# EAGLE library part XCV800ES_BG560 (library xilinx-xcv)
xcv800es_bg560 edit this description Auto generated by make-symbol-device-package-bsdl.ulp Rev. 26 Source: xcv800es_bg560.bsd
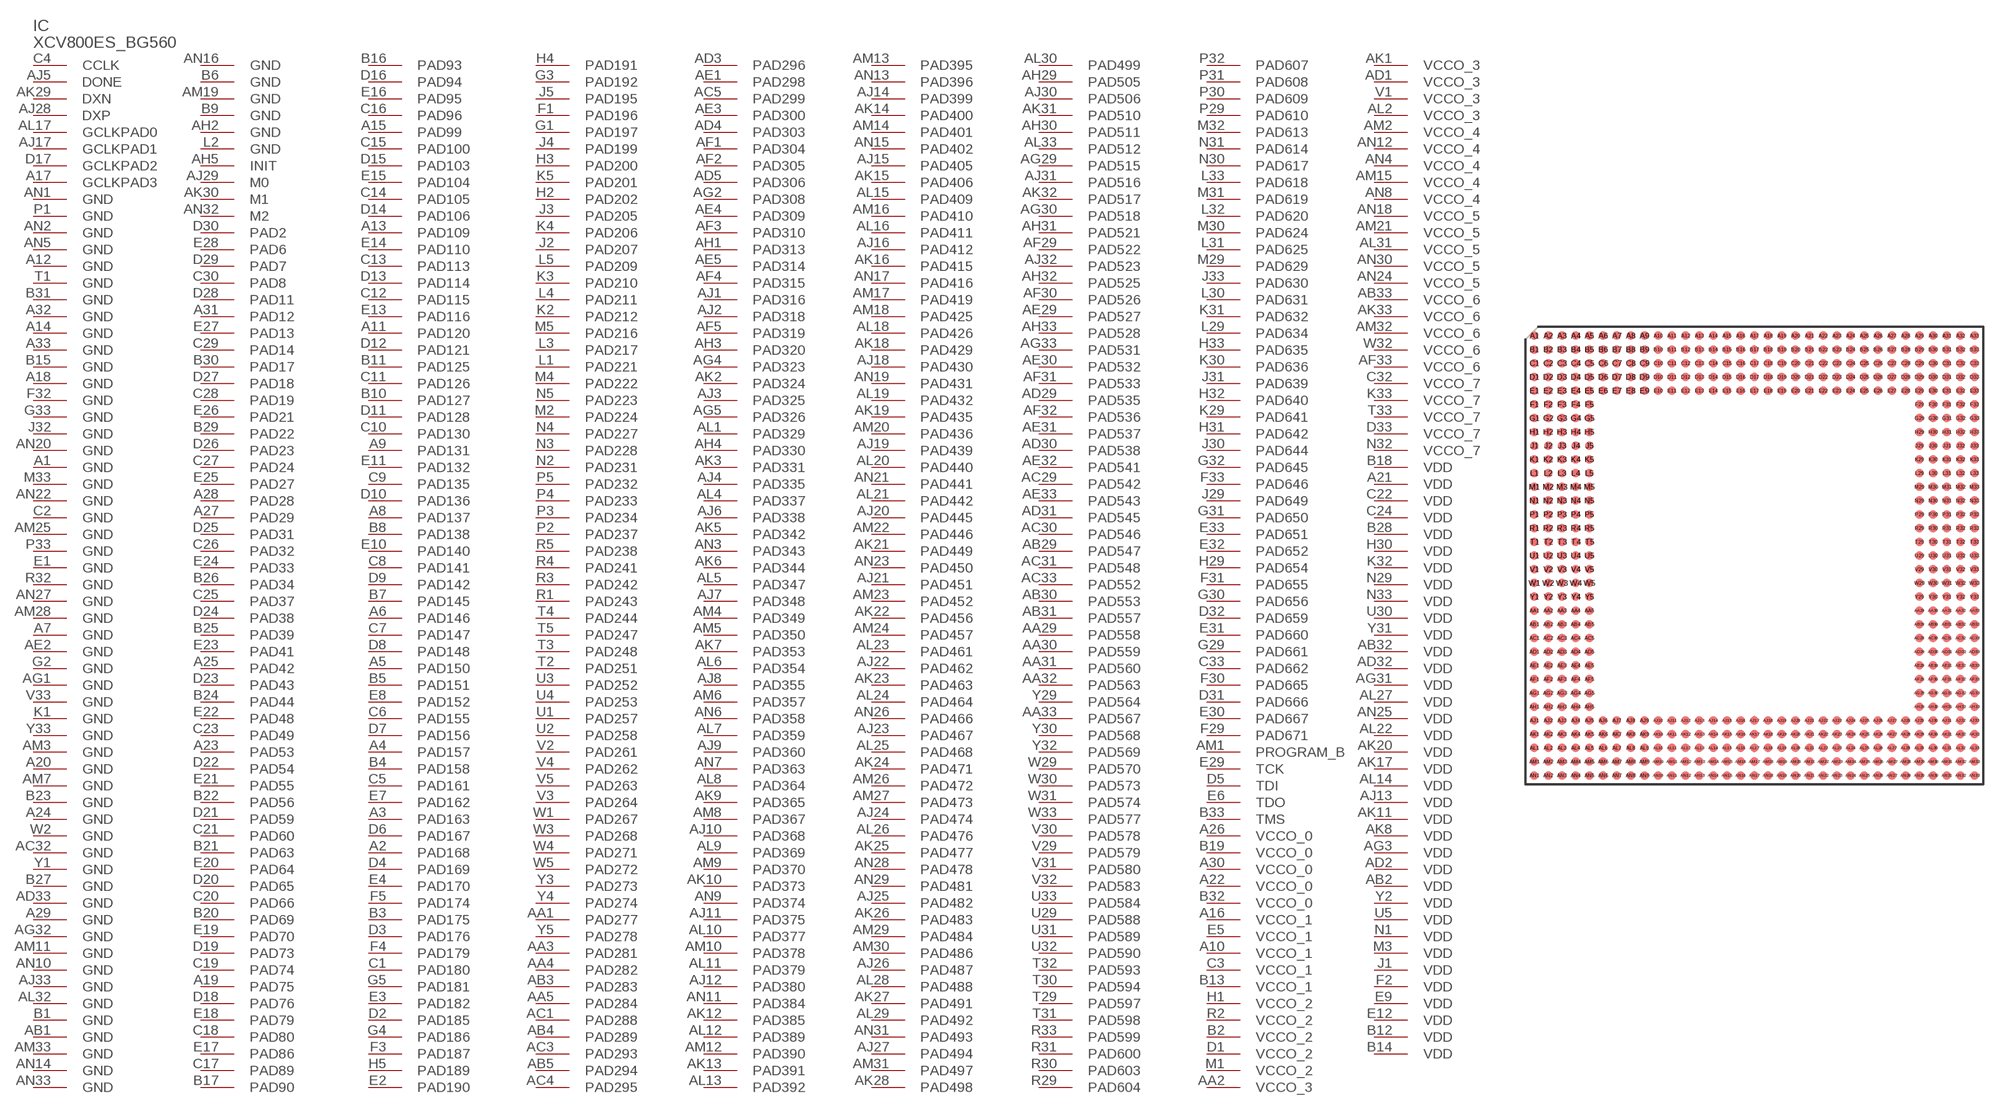
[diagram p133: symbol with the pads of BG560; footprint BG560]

Designator prefix IC

## XCV800ES_BG560 (OC_FARNELL: unknown; OC_NEWARK: unknown)  [BG560]
A1  GND  pwr
A2  PAD168
A3  PAD163
A4  PAD157
A5  PAD150
A6  PAD146
A7  GND  pwr
A8  PAD137
A9  PAD131
A10  VCCO_1  pwr
A11  PAD120
A12  GND  pwr
A13  PAD109
A14  GND  pwr
A15  PAD99
A16  VCCO_1  pwr
A17  GCLKPAD3  in
A18  GND  pwr
A19  PAD75
A20  GND  pwr
A21  VDD  pwr
A22  VCCO_0  pwr
A23  PAD53
A24  GND  pwr
A25  PAD42
A26  VCCO_0  pwr
A27  PAD29
A28  PAD28
A29  GND  pwr
A30  VCCO_0  pwr
A31  PAD12
A32  GND  pwr
A33  GND  pwr
AA1  PAD277
AA2  VCCO_3  pwr
AA3  PAD281
AA4  PAD282
AA5  PAD284
AA29  PAD558
AA30  PAD559
AA31  PAD560
AA32  PAD563
AA33  PAD567
AB1  GND  pwr
AB2  VDD  pwr
AB3  PAD283
AB4  PAD289
AB5  PAD294
AB29  PAD547
AB30  PAD553
AB31  PAD557
AB32  VDD  pwr
AB33  VCCO_6  pwr
AC1  PAD288
AC3  PAD293
AC4  PAD295
AC5  PAD299
AC29  PAD542
AC30  PAD546
AC31  PAD548
AC32  GND  pwr
AC33  PAD552
AD1  VCCO_3  pwr
AD2  VDD  pwr
AD3  PAD296
AD4  PAD303
AD5  PAD306
AD29  PAD535
AD30  PAD538
AD31  PAD545
AD32  VDD  pwr
AD33  GND  pwr
AE1  PAD298
AE2  GND  pwr
AE3  PAD300
AE4  PAD309
AE5  PAD314
AE29  PAD527
AE30  PAD532
AE31  PAD537
AE32  PAD541
AE33  PAD543
AF1  PAD304
AF2  PAD305
AF3  PAD310
AF4  PAD315
AF5  PAD319
AF29  PAD522
AF30  PAD526
AF31  PAD533
AF32  PAD536
AF33  VCCO_6  pwr
AG1  GND  pwr
AG2  PAD308
AG3  VDD  pwr
AG4  PAD323
AG5  PAD326
AG29  PAD515
AG30  PAD518
AG31  VDD  pwr
AG32  GND  pwr
AG33  PAD531
AH1  PAD313
AH2  GND  pwr
AH3  PAD320
AH4  PAD330
AH5  INIT
AH29  PAD505
AH30  PAD511
AH31  PAD521
AH32  PAD525
AH33  PAD528
AJ1  PAD316
AJ2  PAD318
AJ3  PAD325
AJ4  PAD335
AJ5  DONE
AJ6  PAD338
AJ7  PAD348
AJ8  PAD355
AJ9  PAD360
AJ10  PAD368
AJ11  PAD375
AJ12  PAD380
AJ13  VDD  pwr
AJ14  PAD399
AJ15  PAD405
AJ16  PAD412
AJ17  GCLKPAD1  in
AJ18  PAD430
AJ19  PAD439
AJ20  PAD445
AJ21  PAD451
AJ22  PAD462
AJ23  PAD467
AJ24  PAD474
AJ25  PAD482
AJ26  PAD487
AJ27  PAD494
AJ28  DXP  pas
AJ29  M0  in
AJ30  PAD506
AJ31  PAD516
AJ32  PAD523
AJ33  GND  pwr
AK1  VCCO_3  pwr
AK2  PAD324
AK3  PAD331
AK5  PAD342
AK6  PAD344
AK7  PAD353
AK8  VDD  pwr
AK9  PAD365
AK10  PAD373
AK11  VDD  pwr
AK12  PAD385
AK13  PAD391
AK14  PAD400
AK15  PAD406
AK16  PAD415
AK17  VDD  pwr
AK18  PAD429
AK19  PAD435
AK20  VDD  pwr
AK21  PAD449
AK22  PAD456
AK23  PAD463
AK24  PAD471
AK25  PAD477
AK26  PAD483
AK27  PAD491
AK28  PAD498
AK29  DXN  pas
AK30  M1  in
AK31  PAD510
AK32  PAD517
AK33  VCCO_6  pwr
AL1  PAD329
AL2  VCCO_3  pwr
AL4  PAD337
AL5  PAD347
AL6  PAD354
AL7  PAD359
AL8  PAD364
AL9  PAD369
AL10  PAD377
AL11  PAD379
AL12  PAD389
AL13  PAD392
AL14  VDD  pwr
AL15  PAD409
AL16  PAD411
AL17  GCLKPAD0  in
AL18  PAD426
AL19  PAD432
AL20  PAD440
AL21  PAD442
AL22  VDD  pwr
AL23  PAD461
AL24  PAD464
AL25  PAD468
AL26  PAD476
AL27  VDD  pwr
AL28  PAD488
AL29  PAD492
AL30  PAD499
AL31  VCCO_5  pwr
AL32  GND  pwr
AL33  PAD512
AM1  PROGRAM_B  in
AM2  VCCO_4  pwr
AM3  GND  pwr
AM4  PAD349
AM5  PAD350
AM6  PAD357
AM7  GND  pwr
AM8  PAD367
AM9  PAD370
AM10  PAD378
AM11  GND  pwr
AM12  PAD390
AM13  PAD395
AM14  PAD401
AM15  VCCO_4  pwr
AM16  PAD410
AM17  PAD419
AM18  PAD425
AM19  GND  pwr
AM20  PAD436
AM21  VCCO_5  pwr
AM22  PAD446
AM23  PAD452
AM24  PAD457
AM25  GND  pwr
AM26  PAD472
AM27  PAD473
AM28  GND  pwr
AM29  PAD484
AM30  PAD486
AM31  PAD497
AM32  VCCO_6  pwr
AM33  GND  pwr
AN1  GND  pwr
AN2  GND  pwr
AN3  PAD343
AN4  VCCO_4  pwr
AN5  GND  pwr
AN6  PAD358
AN7  PAD363
AN8  VCCO_4  pwr
AN9  PAD374
AN10  GND  pwr
AN11  PAD384
AN12  VCCO_4  pwr
AN13  PAD396
AN14  GND  pwr
AN15  PAD402
AN16  GND  pwr
AN17  PAD416
AN18  VCCO_5  pwr
AN19  PAD431
AN20  GND  pwr
AN21  PAD441
AN22  GND  pwr
AN23  PAD450
AN24  VCCO_5  pwr
AN25  VDD  pwr
AN26  PAD466
AN27  GND  pwr
AN28  PAD478
AN29  PAD481
AN30  VCCO_5  pwr
AN31  PAD493
AN32  M2  in
AN33  GND  pwr
B1  GND  pwr
B2  VCCO_2  pwr
B3  PAD175
B4  PAD158
B5  PAD151
B6  GND  pwr
B7  PAD145
B8  PAD138
B9  GND  pwr
B10  PAD127
B11  PAD125
B12  VDD  pwr
B13  VCCO_1  pwr
B14  VDD  pwr
B15  GND  pwr
B16  PAD93
B17  PAD90
B18  VDD  pwr
B19  VCCO_0  pwr
B20  PAD69
B21  PAD63
B22  PAD56
B23  GND  pwr
B24  PAD44
B25  PAD39
B26  PAD34
B27  GND  pwr
B28  VDD  pwr
B29  PAD22
B30  PAD17
B31  GND  pwr
B32  VCCO_0  pwr
B33  TMS  in
C1  PAD180
C2  GND  pwr
C3  VCCO_1  pwr
C4  CCLK
C5  PAD161
C6  PAD155
C7  PAD147
C8  PAD141
C9  PAD135
C10  PAD130
C11  PAD126
C12  PAD115
C13  PAD113
C14  PAD105
C15  PAD100
C16  PAD96
C17  PAD89
C18  PAD80
C19  PAD74
C20  PAD66
C21  PAD60
C22  VDD  pwr
C23  PAD49
C24  VDD  pwr
C25  PAD37
C26  PAD32
C27  PAD24
C28  PAD19
C29  PAD14
C30  PAD8
C32  VCCO_7  pwr
C33  PAD662
D1  VCCO_2  pwr
D2  PAD185
D3  PAD176
D4  PAD169
D5  TDI  in
D6  PAD167
D7  PAD156
D8  PAD148
D9  PAD142
D10  PAD136
D11  PAD128
D12  PAD121
D13  PAD114
D14  PAD106
D15  PAD103
D16  PAD94
D17  GCLKPAD2  in
D18  PAD76
D19  PAD73
D20  PAD65
D21  PAD59
D22  PAD54
D23  PAD43
D24  PAD38
D25  PAD31
D26  PAD23
D27  PAD18
D28  PAD11
D29  PAD7
D30  PAD2
D31  PAD666
D32  PAD659
D33  VCCO_7  pwr
E1  GND  pwr
E2  PAD190
E3  PAD182
E4  PAD170
E5  VCCO_1  pwr
E6  TDO  out
E7  PAD162
E8  PAD152
E9  VDD  pwr
E10  PAD140
E11  PAD132
E12  VDD  pwr
E13  PAD116
E14  PAD110
E15  PAD104
E16  PAD95
E17  PAD86
E18  PAD79
E19  PAD70
E20  PAD64
E21  PAD55
E22  PAD48
E23  PAD41
E24  PAD33
E25  PAD27
E26  PAD21
E27  PAD13
E28  PAD6
E29  TCK  in
E30  PAD667
E31  PAD660
E32  PAD652
E33  PAD651
F1  PAD196
F2  VDD  pwr
F3  PAD187
F4  PAD179
F5  PAD174
F29  PAD671
F30  PAD665
F31  PAD655
F32  GND  pwr
F33  PAD646
G1  PAD197
G2  GND  pwr
G3  PAD192
G4  PAD186
G5  PAD181
G29  PAD661
G30  PAD656
G31  PAD650
G32  PAD645
G33  GND  pwr
H1  VCCO_2  pwr
H2  PAD202
H3  PAD200
H4  PAD191
H5  PAD189
H29  PAD654
H30  VDD  pwr
H31  PAD642
H32  PAD640
H33  PAD635
J1  VDD  pwr
J2  PAD207
J3  PAD205
J4  PAD199
J5  PAD195
J29  PAD649
J30  PAD644
J31  PAD639
J32  GND  pwr
J33  PAD630
K1  GND  pwr
K2  PAD212
K3  PAD210
K4  PAD206
K5  PAD201
K29  PAD641
K30  PAD636
K31  PAD632
K32  VDD  pwr
K33  VCCO_7  pwr
L1  PAD221
L2  GND  pwr
L3  PAD217
L4  PAD211
L5  PAD209
L29  PAD634
L30  PAD631
L31  PAD625
L32  PAD620
L33  PAD618
M1  VCCO_2  pwr
M2  PAD224
M3  VDD  pwr
M4  PAD222
M5  PAD216
M29  PAD629
M30  PAD624
M31  PAD619
M32  PAD613
M33  GND  pwr
N1  VDD  pwr
N2  PAD231
N3  PAD228
N4  PAD227
N5  PAD223
N29  VDD  pwr
N30  PAD617
N31  PAD614
N32  VCCO_7  pwr
N33  VDD  pwr
P1  GND  pwr
P2  PAD237
P3  PAD234
P4  PAD233
P5  PAD232
P29  PAD610
P30  PAD609
P31  PAD608
P32  PAD607
P33  GND  pwr
R1  PAD243
R2  VCCO_2  pwr
R3  PAD242
R4  PAD241
R5  PAD238
R29  PAD604
R30  PAD603
R31  PAD600
R32  GND  pwr
R33  PAD599
T1  GND  pwr
T2  PAD251
T3  PAD248
T4  PAD244
T5  PAD247
T29  PAD597
T30  PAD594
T31  PAD598
T32  PAD593
T33  VCCO_7  pwr
U1  PAD257
U2  PAD258
U3  PAD252
U4  PAD253
U5  VDD  pwr
U29  PAD588
U30  VDD  pwr
U31  PAD589
U32  PAD590
U33  PAD584
V1  VCCO_3  pwr
V2  PAD261
V3  PAD264
V4  PAD262
V5  PAD263
V29  PAD579
V30  PAD578
V31  PAD580
V32  PAD583
V33  GND  pwr
W1  PAD267
W2  GND  pwr
W3  PAD268
W4  PAD271
W5  PAD272
W29  PAD570
W30  PAD573
W31  PAD574
W32  VCCO_6  pwr
W33  PAD577
Y1  GND  pwr
Y2  VDD  pwr
Y3  PAD273
Y4  PAD274
Y5  PAD278
Y29  PAD564
Y30  PAD568
Y31  VDD  pwr
Y32  PAD569
Y33  GND  pwr

## Footprint BG560 (pad centres in mm)
Metal BGA (BG560) Auto generated by make-symbol-device-package-bsdl.ulp Rev. 26 Source: xcv1000_bg560_1532.bsd; bg560.pdf
smd 0.8 x 0.8: A1 -20.32,20.32; A2 -19.05,20.32; A3 -17.78,20.32; A4 -16.51,20.32; A5 -15.24,20.32; A6 -13.97,20.32; A7 -12.7,20.32; A8 -11.43,20.32; A9 -10.16,20.32; A10 -8.89,20.32; A11 -7.62,20.32; A12 -6.35,20.32; A13 -5.08,20.32; A14 -3.81,20.32; A15 -2.54,20.32; A16 -1.27,20.32; A17 0,20.32; A18 1.27,20.32; A19 2.54,20.32; A20 3.81,20.32; A21 5.08,20.32; A22 6.35,20.32; A23 7.62,20.32; A24 8.89,20.32; A25 10.16,20.32; A26 11.43,20.32; A27 12.7,20.32; A28 13.97,20.32; A29 15.24,20.32; A30 16.51,20.32; A31 17.78,20.32; A32 19.05,20.32; A33 20.32,20.32; AA1 -20.32,-5.08; AA2 -19.05,-5.08; AA3 -17.78,-5.08; AA4 -16.51,-5.08; AA5 -15.24,-5.08; AA29 15.24,-5.08; AA30 16.51,-5.08; AA31 17.78,-5.08; AA32 19.05,-5.08; AA33 20.32,-5.08; AB1 -20.32,-6.35; AB2 -19.05,-6.35; AB3 -17.78,-6.35; AB4 -16.51,-6.35; AB5 -15.24,-6.35; AB29 15.24,-6.35; AB30 16.51,-6.35; AB31 17.78,-6.35; AB32 19.05,-6.35; AB33 20.32,-6.35; AC1 -20.32,-7.62; AC2 -19.05,-7.62; AC3 -17.78,-7.62; AC4 -16.51,-7.62; AC5 -15.24,-7.62; AC29 15.24,-7.62; AC30 16.51,-7.62; AC31 17.78,-7.62; AC32 19.05,-7.62; AC33 20.32,-7.62; AD1 -20.32,-8.89; AD2 -19.05,-8.89; AD3 -17.78,-8.89; AD4 -16.51,-8.89; AD5 -15.24,-8.89; AD29 15.24,-8.89; AD30 16.51,-8.89; AD31 17.78,-8.89; AD32 19.05,-8.89; AD33 20.32,-8.89; AE1 -20.32,-10.16; AE2 -19.05,-10.16; AE3 -17.78,-10.16; AE4 -16.51,-10.16; AE5 -15.24,-10.16; AE29 15.24,-10.16; AE30 16.51,-10.16; AE31 17.78,-10.16; AE32 19.05,-10.16; AE33 20.32,-10.16; AF1 -20.32,-11.43; AF2 -19.05,-11.43; AF3 -17.78,-11.43; AF4 -16.51,-11.43; AF5 -15.24,-11.43; AF29 15.24,-11.43; AF30 16.51,-11.43; AF31 17.78,-11.43; AF32 19.05,-11.43; AF33 20.32,-11.43; AG1 -20.32,-12.7; AG2 -19.05,-12.7; AG3 -17.78,-12.7; AG4 -16.51,-12.7; AG5 -15.24,-12.7; AG29 15.24,-12.7; AG30 16.51,-12.7; AG31 17.78,-12.7; AG32 19.05,-12.7; AG33 20.32,-12.7; AH1 -20.32,-13.97; AH2 -19.05,-13.97; AH3 -17.78,-13.97; AH4 -16.51,-13.97; AH5 -15.24,-13.97; AH29 15.24,-13.97; AH30 16.51,-13.97; AH31 17.78,-13.97; AH32 19.05,-13.97; AH33 20.32,-13.97; AJ1 -20.32,-15.24; AJ2 -19.05,-15.24; AJ3 -17.78,-15.24; AJ4 -16.51,-15.24; AJ5 -15.24,-15.24; AJ6 -13.97,-15.24; AJ7 -12.7,-15.24; AJ8 -11.43,-15.24; AJ9 -10.16,-15.24; AJ10 -8.89,-15.24; AJ11 -7.62,-15.24; AJ12 -6.35,-15.24; AJ13 -5.08,-15.24; AJ14 -3.81,-15.24; AJ15 -2.54,-15.24; AJ16 -1.27,-15.24; AJ17 0,-15.24; AJ18 1.27,-15.24; AJ19 2.54,-15.24; AJ20 3.81,-15.24; AJ21 5.08,-15.24; AJ22 6.35,-15.24; AJ23 7.62,-15.24; AJ24 8.89,-15.24; AJ25 10.16,-15.24; AJ26 11.43,-15.24; AJ27 12.7,-15.24; AJ28 13.97,-15.24; AJ29 15.24,-15.24; AJ30 16.51,-15.24; AJ31 17.78,-15.24; AJ32 19.05,-15.24; AJ33 20.32,-15.24; AK1 -20.32,-16.51; AK2 -19.05,-16.51; AK3 -17.78,-16.51; AK4 -16.51,-16.51; AK5 -15.24,-16.51; AK6 -13.97,-16.51; AK7 -12.7,-16.51; AK8 -11.43,-16.51; AK9 -10.16,-16.51; AK10 -8.89,-16.51; AK11 -7.62,-16.51; AK12 -6.35,-16.51; AK13 -5.08,-16.51; AK14 -3.81,-16.51; AK15 -2.54,-16.51; AK16 -1.27,-16.51; AK17 0,-16.51; AK18 1.27,-16.51; AK19 2.54,-16.51; AK20 3.81,-16.51; AK21 5.08,-16.51; AK22 6.35,-16.51; AK23 7.62,-16.51; AK24 8.89,-16.51; AK25 10.16,-16.51; AK26 11.43,-16.51; AK27 12.7,-16.51; AK28 13.97,-16.51; AK29 15.24,-16.51; AK30 16.51,-16.51; AK31 17.78,-16.51; AK32 19.05,-16.51; AK33 20.32,-16.51; AL1 -20.32,-17.78; AL2 -19.05,-17.78; AL3 -17.78,-17.78; AL4 -16.51,-17.78; AL5 -15.24,-17.78; AL6 -13.97,-17.78; AL7 -12.7,-17.78; AL8 -11.43,-17.78; AL9 -10.16,-17.78; AL10 -8.89,-17.78; AL11 -7.62,-17.78; AL12 -6.35,-17.78; AL13 -5.08,-17.78; AL14 -3.81,-17.78; AL15 -2.54,-17.78; AL16 -1.27,-17.78; AL17 0,-17.78; AL18 1.27,-17.78; AL19 2.54,-17.78; AL20 3.81,-17.78; AL21 5.08,-17.78; AL22 6.35,-17.78; AL23 7.62,-17.78; AL24 8.89,-17.78; AL25 10.16,-17.78; AL26 11.43,-17.78; AL27 12.7,-17.78; AL28 13.97,-17.78; AL29 15.24,-17.78; AL30 16.51,-17.78; AL31 17.78,-17.78; AL32 19.05,-17.78; AL33 20.32,-17.78; AM1 -20.32,-19.05; AM2 -19.05,-19.05; AM3 -17.78,-19.05; AM4 -16.51,-19.05; AM5 -15.24,-19.05; AM6 -13.97,-19.05; AM7 -12.7,-19.05; AM8 -11.43,-19.05; AM9 -10.16,-19.05; AM10 -8.89,-19.05; AM11 -7.62,-19.05; AM12 -6.35,-19.05; AM13 -5.08,-19.05; AM14 -3.81,-19.05; AM15 -2.54,-19.05; AM16 -1.27,-19.05; AM17 0,-19.05; AM18 1.27,-19.05; AM19 2.54,-19.05; AM20 3.81,-19.05; AM21 5.08,-19.05; AM22 6.35,-19.05; AM23 7.62,-19.05; AM24 8.89,-19.05; AM25 10.16,-19.05; AM26 11.43,-19.05; AM27 12.7,-19.05; AM28 13.97,-19.05; AM29 15.24,-19.05; AM30 16.51,-19.05; AM31 17.78,-19.05; AM32 19.05,-19.05; AM33 20.32,-19.05; AN1 -20.32,-20.32; AN2 -19.05,-20.32; AN3 -17.78,-20.32; AN4 -16.51,-20.32; AN5 -15.24,-20.32; AN6 -13.97,-20.32; AN7 -12.7,-20.32; AN8 -11.43,-20.32; AN9 -10.16,-20.32; AN10 -8.89,-20.32; AN11 -7.62,-20.32; AN12 -6.35,-20.32; AN13 -5.08,-20.32; AN14 -3.81,-20.32; AN15 -2.54,-20.32; AN16 -1.27,-20.32; AN17 0,-20.32; AN18 1.27,-20.32; AN19 2.54,-20.32; AN20 3.81,-20.32; AN21 5.08,-20.32; AN22 6.35,-20.32; AN23 7.62,-20.32; AN24 8.89,-20.32; AN25 10.16,-20.32; AN26 11.43,-20.32; AN27 12.7,-20.32; AN28 13.97,-20.32; AN29 15.24,-20.32; AN30 16.51,-20.32; AN31 17.78,-20.32; AN32 19.05,-20.32; AN33 20.32,-20.32; B1 -20.32,19.05; B2 -19.05,19.05; B3 -17.78,19.05; B4 -16.51,19.05; B5 -15.24,19.05; B6 -13.97,19.05; B7 -12.7,19.05; B8 -11.43,19.05; B9 -10.16,19.05; B10 -8.89,19.05; B11 -7.62,19.05; B12 -6.35,19.05; B13 -5.08,19.05; B14 -3.81,19.05; B15 -2.54,19.05; B16 -1.27,19.05; B17 0,19.05; B18 1.27,19.05; B19 2.54,19.05; B20 3.81,19.05; B21 5.08,19.05; B22 6.35,19.05; B23 7.62,19.05; B24 8.89,19.05; B25 10.16,19.05; B26 11.43,19.05; B27 12.7,19.05; B28 13.97,19.05; B29 15.24,19.05; B30 16.51,19.05; B31 17.78,19.05; B32 19.05,19.05; B33 20.32,19.05; C1 -20.32,17.78; C2 -19.05,17.78; C3 -17.78,17.78; C4 -16.51,17.78; C5 -15.24,17.78; C6 -13.97,17.78; C7 -12.7,17.78; C8 -11.43,17.78; C9 -10.16,17.78; C10 -8.89,17.78; C11 -7.62,17.78; C12 -6.35,17.78; C13 -5.08,17.78; C14 -3.81,17.78; C15 -2.54,17.78; C16 -1.27,17.78; C17 0,17.78; C18 1.27,17.78; C19 2.54,17.78; C20 3.81,17.78; C21 5.08,17.78; C22 6.35,17.78; C23 7.62,17.78; C24 8.89,17.78; C25 10.16,17.78; C26 11.43,17.78; C27 12.7,17.78; C28 13.97,17.78; C29 15.24,17.78; C30 16.51,17.78; C31 17.78,17.78; C32 19.05,17.78; C33 20.32,17.78; D1 -20.32,16.51; D2 -19.05,16.51; D3 -17.78,16.51; D4 -16.51,16.51; D5 -15.24,16.51; D6 -13.97,16.51; D7 -12.7,16.51; D8 -11.43,16.51; D9 -10.16,16.51; D10 -8.89,16.51; D11 -7.62,16.51; D12 -6.35,16.51; D13 -5.08,16.51; D14 -3.81,16.51; D15 -2.54,16.51; D16 -1.27,16.51; D17 0,16.51; D18 1.27,16.51; D19 2.54,16.51; D20 3.81,16.51; D21 5.08,16.51; D22 6.35,16.51; D23 7.62,16.51; D24 8.89,16.51; D25 10.16,16.51; D26 11.43,16.51; D27 12.7,16.51; D28 13.97,16.51; D29 15.24,16.51; D30 16.51,16.51; D31 17.78,16.51; D32 19.05,16.51; D33 20.32,16.51; E1 -20.32,15.24; E2 -19.05,15.24; E3 -17.78,15.24; E4 -16.51,15.24; E5 -15.24,15.24; E6 -13.97,15.24; E7 -12.7,15.24; E8 -11.43,15.24; E9 -10.16,15.24; E10 -8.89,15.24; E11 -7.62,15.24; E12 -6.35,15.24; E13 -5.08,15.24; E14 -3.81,15.24; E15 -2.54,15.24; E16 -1.27,15.24; E17 0,15.24; E18 1.27,15.24; E19 2.54,15.24; E20 3.81,15.24; E21 5.08,15.24; E22 6.35,15.24; E23 7.62,15.24; E24 8.89,15.24; E25 10.16,15.24; E26 11.43,15.24; E27 12.7,15.24; E28 13.97,15.24; E29 15.24,15.24; E30 16.51,15.24; E31 17.78,15.24; E32 19.05,15.24; E33 20.32,15.24; F1 -20.32,13.97; F2 -19.05,13.97; F3 -17.78,13.97; F4 -16.51,13.97; F5 -15.24,13.97; F29 15.24,13.97; F30 16.51,13.97; F31 17.78,13.97; F32 19.05,13.97; F33 20.32,13.97; G1 -20.32,12.7; G2 -19.05,12.7; G3 -17.78,12.7; G4 -16.51,12.7; G5 -15.24,12.7; G29 15.24,12.7; G30 16.51,12.7; G31 17.78,12.7; G32 19.05,12.7; G33 20.32,12.7; H1 -20.32,11.43; H2 -19.05,11.43; H3 -17.78,11.43; H4 -16.51,11.43; H5 -15.24,11.43; H29 15.24,11.43; H30 16.51,11.43; H31 17.78,11.43; H32 19.05,11.43; H33 20.32,11.43; J1 -20.32,10.16; J2 -19.05,10.16; J3 -17.78,10.16; J4 -16.51,10.16; J5 -15.24,10.16; J29 15.24,10.16; J30 16.51,10.16; J31 17.78,10.16; J32 19.05,10.16; J33 20.32,10.16; K1 -20.32,8.89; K2 -19.05,8.89; K3 -17.78,8.89; K4 -16.51,8.89; K5 -15.24,8.89; K29 15.24,8.89; K30 16.51,8.89; K31 17.78,8.89; K32 19.05,8.89; K33 20.32,8.89; L1 -20.32,7.62; L2 -19.05,7.62; L3 -17.78,7.62; L4 -16.51,7.62; L5 -15.24,7.62; L29 15.24,7.62; L30 16.51,7.62; L31 17.78,7.62; L32 19.05,7.62; L33 20.32,7.62; M1 -20.32,6.35; M2 -19.05,6.35; M3 -17.78,6.35; M4 -16.51,6.35; M5 -15.24,6.35; M29 15.24,6.35; M30 16.51,6.35; M31 17.78,6.35; M32 19.05,6.35; M33 20.32,6.35; N1 -20.32,5.08; N2 -19.05,5.08; N3 -17.78,5.08; N4 -16.51,5.08; N5 -15.24,5.08; N29 15.24,5.08; N30 16.51,5.08; N31 17.78,5.08; N32 19.05,5.08; N33 20.32,5.08; P1 -20.32,3.81; P2 -19.05,3.81; P3 -17.78,3.81; P4 -16.51,3.81; P5 -15.24,3.81; P29 15.24,3.81; P30 16.51,3.81; P31 17.78,3.81; P32 19.05,3.81; P33 20.32,3.81; R1 -20.32,2.54; R2 -19.05,2.54; R3 -17.78,2.54; R4 -16.51,2.54; R5 -15.24,2.54; R29 15.24,2.54; R30 16.51,2.54; R31 17.78,2.54; R32 19.05,2.54; R33 20.32,2.54; T1 -20.32,1.27; T2 -19.05,1.27; T3 -17.78,1.27; T4 -16.51,1.27; T5 -15.24,1.27; T29 15.24,1.27; T30 16.51,1.27; T31 17.78,1.27; T32 19.05,1.27; T33 20.32,1.27; U1 -20.32,0; U2 -19.05,0; U3 -17.78,0; U4 -16.51,0; U5 -15.24,0; U29 15.24,0; U30 16.51,0; U31 17.78,0; U32 19.05,0; U33 20.32,0; V1 -20.32,-1.27; V2 -19.05,-1.27; V3 -17.78,-1.27; V4 -16.51,-1.27; V5 -15.24,-1.27; V29 15.24,-1.27; V30 16.51,-1.27; V31 17.78,-1.27; V32 19.05,-1.27; V33 20.32,-1.27; W1 -20.32,-2.54; W2 -19.05,-2.54; W3 -17.78,-2.54; W4 -16.51,-2.54; W5 -15.24,-2.54; W29 15.24,-2.54; W30 16.51,-2.54; W31 17.78,-2.54; W32 19.05,-2.54; W33 20.32,-2.54; Y1 -20.32,-3.81; Y2 -19.05,-3.81; Y3 -17.78,-3.81; Y4 -16.51,-3.81; Y5 -15.24,-3.81; Y29 15.24,-3.81; Y30 16.51,-3.81; Y31 17.78,-3.81; Y32 19.05,-3.81; Y33 20.32,-3.81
